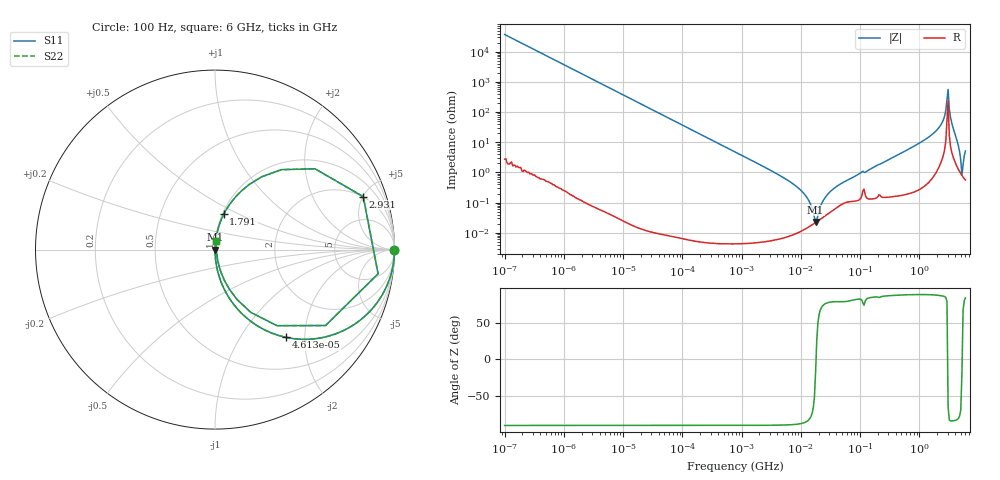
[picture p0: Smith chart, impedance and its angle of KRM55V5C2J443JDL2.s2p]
!Murata Part Number: KRM55V5C2J443JDL2
!These Parameters are Measured in Series Mode Connection
!Data Generated on Jan 08, 2026
!  o--ll--o
!Port1  Port2
!  o------o
!Operation Temp=25[degC], DC Bias Voltage=0[V]
!Freq. Start=100[Hz] Stop=6[GHz] 401[Steps]
# Hz S RI R 50
!Freq.(Hz) S11(Real) S11(Imag) S21(Real) S21(Imag) S12(Real) S12(Imag) S22(Real) S22(Imag)
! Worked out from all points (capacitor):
!   401 points, 100 Hz to 6 GHz, reference 50 ohm
!   read as one part in series: C = 42.7 nF near 109 Hz
!   lowest |Z| = 22.8 mohm at 17.79 MHz (marker M1)
!   series resonance near 18.08 MHz, so ESL is about 1.8 nH
!   S11 on the Smith chart (normalised r, x): 100 Hz: open; 46.13 kHz: 1.00, -1.62; 1.791 GHz: 1.02, +0.42; 2.931 GHz: 1.97, +5.03; 6 GHz: 1.01, +0.10
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100  1 -0.00268  7.4e-06 0.00268  7.4e-06 0.00268  1 -0.00268
2008  0.9971 -0.0537  0.0029 0.0537  0.0029 0.0537  0.9971 -0.0537
12592  0.8975 -0.3032  0.1025 0.3032  0.1025 0.3032  0.8975 -0.3032
40335  0.4606 -0.4984  0.5394 0.4984  0.5394 0.4984  0.4606 -0.4984
46134  0.3949 -0.4888  0.6051 0.4888  0.6051 0.4888  0.3949 -0.4888
129199  0.0769 -0.2663  0.9231 0.2663  0.9231 0.2663  0.0769 -0.2663
774597  0.00234 -0.0479  0.9977 0.0479  0.9977 0.0479  0.00234 -0.0479
7599586  0.000103 -0.00401  0.9999 0.00401  0.9999 0.00401  0.000103 -0.00401
1.189169e7  0.000136 -0.00176  0.9999 0.00176  0.9999 0.00176  0.000136 -0.00176
1.555665e7  0.000184 -0.000609  0.9998 0.000609  0.9998 0.000609  0.000184 -0.000609
1.779312e7  0.000219 -6.31e-05  0.9998 6.31e-05  0.9998 6.31e-05  0.000219 -6.31e-05
2.545746e7  0.000359 0.00138  0.9996 -0.00138  0.9996 -0.00138  0.000359 0.00138
3.64232e7  0.000598 0.00291  0.9994 -0.00291  0.9994 -0.00291  0.000598 0.00291
3.124326e8  0.00226 0.0271  0.9977 -0.0271  0.9977 -0.0271  0.00226 0.0271
1.791126e9  0.0486 0.197  0.9514 -0.197  0.9514 -0.197  0.0486 0.197
2.34314e9  0.1479 0.3275  0.8521 -0.3275  0.8521 -0.3275  0.1479 0.3275
2.679998e9  0.3699 0.4455  0.6301 -0.4455  0.6301 -0.4455  0.3699 0.4455
2.931063e9  0.826 0.2949  0.174 -0.2949  0.174 -0.2949  0.826 0.2949
3.505958e9  0.1995 -0.3497  0.8005 0.3497  0.8005 0.3497  0.1995 -0.3497
5.016141e9  0.00956 -0.023  0.9904 0.023  0.9904 0.023  0.00956 -0.023
5.486059e9  0.00722 0.0162  0.9928 -0.0162  0.9928 -0.0162  0.00722 0.0162
6e9  0.00812 0.0503  0.9919 -0.0503  0.9919 -0.0503  0.00812 0.0503
